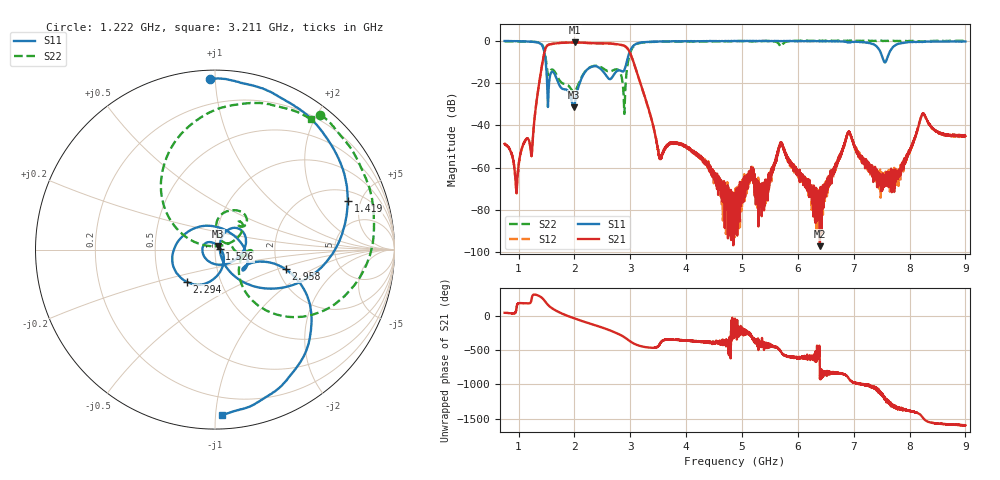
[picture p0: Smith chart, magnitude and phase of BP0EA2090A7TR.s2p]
!Agilent Technologies,E8358A,US41080443,A.07.50.56
!Agilent E8358A: A.07.50.56
!Date: Friday, November 20, 2015 11:11:02
!Correction: S11(Full 2 Port(1,2))
!S21(Full 2 Port(1,2))
!S12(Full 2 Port(1,2))
!S22(Full 2 Port(1,2))
!S2P File: Measurements: S11, S21, S12, S22:
# Hz S  dB  R 50
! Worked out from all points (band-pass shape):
!   6401 points, 750 MHz to 9 GHz, reference 50 ohm
!   highest |S21| = -0.80 dB at 2.004 GHz (marker M1); lowest = -97.3 dB at 6.395 GHz (marker M2)
!   |S21| within 3 dB of the highest: 1.481 GHz to 2.956 GHz (1.475 GHz wide, 66.5 % of centre)
!   lowest |S11| = -31.6 dB at 1.984 GHz (marker M3), VSWR 1.05, Z = 51.8 + j2.02 ohm
!   |S11| at or under -10 dB: 1.486 GHz to 2.937 GHz (1.451 GHz wide, 65.6 % of centre); 7.546841 GHz to 7.572153 GHz (25.31 MHz wide, 0.335 % of centre)
!   |S22| runs from -34.6 to 0.2 dB; largest |S21 - S12| = 0.0066
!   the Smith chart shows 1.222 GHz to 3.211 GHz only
!   S11 on the Smith chart (normalised r, x): 1.222 GHz: 0.05, +0.97; 1.419 GHz: 2.72, +3.85; 1.526 GHz: 1.05, +0.01; 2.294 GHz: 0.69, -0.26; 2.958 GHz: 2.19, -0.58; 3.211 GHz: 0.09, -1.04
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7.5e8  -0.09 143.2  -48.82 39.6  -48.80 39.3  -0.19 116.4
1.221797e9  -0.43 91.6  -52.83 -160.1  -52.82 -159.5  -0.41 52.1
1.419023e9  -2.07 20.0  -11.55 -103.6  -11.59 -103.4  -1.74 -11.3
1.526016e9  -31.36 10.5  -1.97 154.7  -2.02 154.8  -15.99 -31.0
1.672969e9  -17.30 -18.7  -1.16 69.9  -1.20 70.0  -15.83 -11.4
1.983633e9  -31.55 47.5  -0.81 -37.5  -0.85 -37.5  -24.22 46.7
2.004258e9  -29.98 6.6  -0.80 -43.5  -0.85 -43.4  -24.09 58.1
2.12543e9  -17.87 -77.3  -0.87 -77.2  -0.91 -77.2  -17.40 87.2
2.294297e9  -12.42 -131.1  -1.10 -121.4  -1.13 -121.3  -12.36 65.5
2.74418e9  -14.71 -11.8  -1.57 108.4  -1.60 108.5  -13.52 47.0
2.958164e9  -7.78 -15.5  -3.88 8.4  -3.94 8.6  -10.13 145.3
3.21082e9  -0.72 -87.6  -22.47 -89.0  -22.56 -89.1  -0.90 53.8
3.500859e9  -0.35 -122.2  -52.20 -86.1  -52.49 -82.9  -0.43 12.4
4.875e9  -0.10 179.0  -91.43 -45.2  -75.26 153.3  -0.14 -106.0
5.701289e9  -0.09 -178.5  -48.33 -170.8  -48.36 -174.0  -2.63 -147.6
6.25043e9  -0.12 173.5  -69.51 116.3  -71.85 100.8  -0.05 -159.5
6.394805e9  -0.26 171.6  -97.25 -156.1  -79.38 -160.5  0.06 -163.2
6.909141e9  -0.72 155.0  -43.15 169.9  -43.20 169.4  -0.03 -172.4
7.395117e9  -2.31 102.7  -61.99 15.4  -64.48 9.9  -0.02 175.9
7.625859e9  -6.40 -106.6  -69.28 164.5  -66.56 173.7  -0.09 169.0
8.236875e9  -0.52 152.6  -34.51 -41.8  -34.57 -42.3  -0.40 143.9
9e9  -0.36 126.1  -45.02 -155.4  -45.16 -156.9  0.01 111.9
